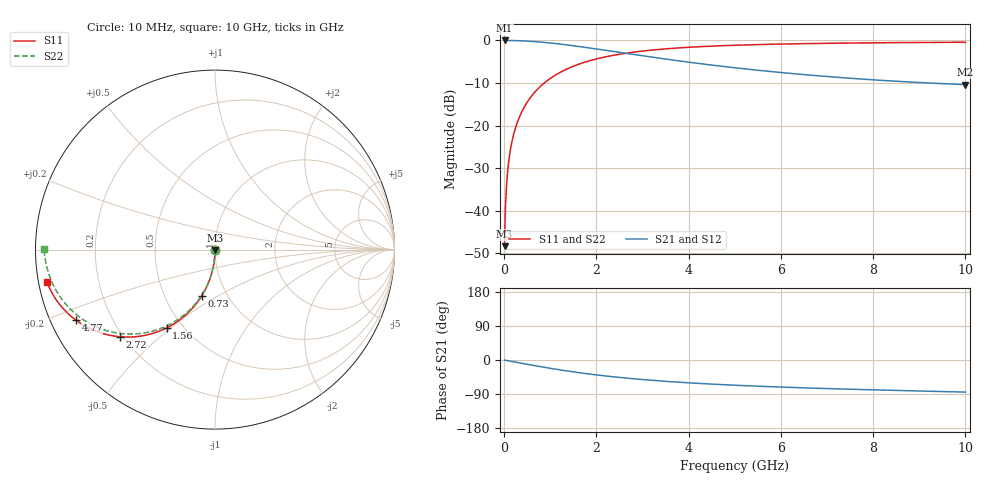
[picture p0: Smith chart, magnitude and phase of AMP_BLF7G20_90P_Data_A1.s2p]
! Created Tue May 08 13:41:25 2012
# ghz S ma R 50
! 2 Port Network Data from SP1.SP block
! freq  magS11  angS11  magS21  angS21  magS12  angS12  magS22  angS22
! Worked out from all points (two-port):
!   1000 points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, 10 MHz to 10 GHz, reference 50 ohm
!   highest |S21| = 0.00 dB at 10 MHz (marker M1); lowest = -10.4 dB at 10 GHz (marker M2)
!   |S21| within 3 dB of the highest: start of sweep to 2.626 GHz
!   lowest |S11| = -48.3 dB at 10 MHz (marker M3), VSWR 1.01, Z = 50 - j0.384 ohm
!   |S11| at or under -10 dB: start of sweep to 868.7 MHz
!   |S22| runs from -48.3 to -0.4 dB; largest |S21 - S12| = 0
!   S11 on the Smith chart (normalised r, x): 10 MHz: 1.00, -0.01; 730 MHz: 0.76, -0.42; 1.56 GHz: 0.41, -0.48; 2.72 GHz: 0.19, -0.38; 4.77 GHz: 0.07, -0.24; 10 GHz: 0.02, -0.10
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0.01  0.003838 -90.2  1 -0.2  1 -0.2  0.003838 -90.2
0.04  0.01536 -90.9  0.9999 -0.9  0.9999 -0.9  0.01536 -90.9
0.07  0.02687 -91.6  0.9996 -1.6  0.9996 -1.6  0.02687 -91.6
0.09  0.03454 -92.0  0.9994 -2.1  0.9994 -2.1  0.03454 -92.1
0.11  0.0422 -92.5  0.9991 -2.5  0.9991 -2.5  0.0422 -92.6
0.14  0.05368 -93.1  0.9985 -3.2  0.9985 -3.2  0.05368 -93.3
0.2  0.07658 -94.5  0.9971 -4.6  0.9971 -4.6  0.07658 -94.7
0.29  0.1107 -96.5  0.9938 -6.6  0.9938 -6.6  0.1107 -96.8
0.41  0.1555 -99.2  0.9878 -9.3  0.9878 -9.3  0.1555 -99.5
0.56  0.2102 -102.4  0.9776 -12.7  0.9776 -12.7  0.2102 -102.9
0.73  0.2698 -106.1  0.9629 -16.4  0.9629 -16.4  0.2698 -106.7
1.1  0.3886 -113.5  0.9214 -23.9  0.9214 -23.9  0.3886 -114.4
1.56  0.5126 -121.7  0.8586 -32.4  0.8586 -32.4  0.5126 -123.0
1.68  0.5406 -123.7  0.8413 -34.4  0.8413 -34.4  0.5406 -125.1
2.16  0.6358 -130.7  0.7718 -41.6  0.7718 -41.6  0.6357 -132.5
2.72  0.7183 -137.5  0.6957 -48.6  0.6957 -48.6  0.7182 -139.7
3.34  0.7831 -143.5  0.6218 -54.9  0.6218 -54.9  0.7831 -146.3
4.77  0.8695 -153.2  0.4938 -65.3  0.4938 -65.3  0.8695 -157.3
5.01  0.8787 -154.4  0.4772 -66.6  0.4772 -66.6  0.8787 -158.8
6.67  0.9208 -161.1  0.39 -74.2  0.39 -74.2  0.9207 -167.2
8.34  0.9418 -165.7  0.3358 -79.8  0.3358 -79.8  0.9418 -174.0
10  0.9529 -169.0  0.3031 -84.7  0.3031 -84.7  0.9528 179.7
